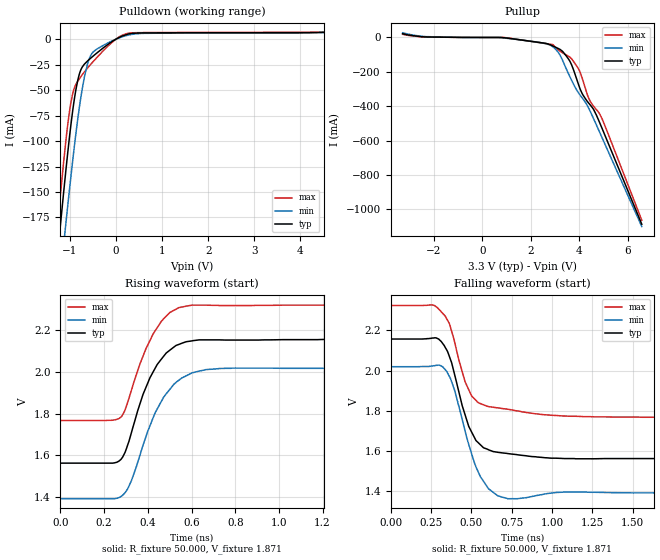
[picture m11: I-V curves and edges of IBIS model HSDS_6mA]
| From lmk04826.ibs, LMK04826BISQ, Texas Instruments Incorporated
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[Model]   HSDS_6mA
Model_type   Output
Polarity   Non-Inverting
Vmeas = 1.9
Vref = 1.9
Cref = 15pF
Rref = 50
|   typ   min   max
|   (nom PVT)   (Fast PVT)   (slow PVT)
C_comp   1.492p   1.392p   1.674p
|C_comp (hi state)   1.492p   1.392p   1.674p
|C_comp (low state)   2.777p   2.419p   2.781p
| Where   nom PVT is  Nominal Process, 3.3V, 27C
|   Fast PVT is Strong Process, 3.45V, -40C
|   Slow PVT is Weak Process, 3.15V, 125C
[Voltage Range]   3.3   3.15   3.45
[Temperature Range]   27   125   -40
[Pullup Reference]   3.3   3.15   3.45
[Pulldown Reference]   0   0   0
[Power Clamp Reference]   3.3   3.15   3.45
[GND Clamp Reference]   0   0   0
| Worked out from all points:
|   slope of the pulldown table from 0 to 0.495 V, typ, clamps not added: 81.8 ohm
|   slope of the pullup table from 0 to 0.495 V, typ, clamps not added: 8 kohm
|   falling waveform, R_fixture 50.000, V_fixture 1.871: 20-80 % time 131ps typ, 131ps min, 127ps max; typ from 2.16 V to 1.56 V
|   rising waveform, R_fixture 50.000, V_fixture 1.871: 20-80 % time 127ps typ, 145ps min, 127ps max; typ from 1.56 V to 2.16 V
[Pulldown]
|   Voltage   I(typ)   I(min)   I(max)
-3.3V     -1.225A    -1.2A      -1.253A
-1.28V    -220mA     -267.9mA   -190.8mA
-1.221V   -191.9mA   -241.5mA   -162.2mA
-1.122V   -146.4mA   -198mA     -116.6mA
-1.073V   -124.5mA   -176.5mA   -95.65mA
-993.3mV  -91.71mA   -143.1mA   -67.69mA
-864.6mV  -49.48mA   -92.41mA   -44.34mA
-755.7mV  -29.9mA    -56.55mA   -36.73mA
-607.2mV  -21.23mA   -23.33mA   -28.05mA
-409.2mV  -13.55mA   -9.712mA   -17.97mA
145.2mV   3.146mA    2.35mA     3.956mA
6.59V     8.158mA    8.228mA    8.143mA
[Pullup]
|   Voltage   I(typ)   I(min)   I(max)
-3.3V     22.29mA    27.13mA    18.75mA
-2.35V    3.194mA    4.974mA    2.65mA
887.7mV   -1.305mA   -2.825mA   -285.8uA
2.363V    -29.22mA   -28.44mA   -30.16mA
2.907V    -48.93mA   -53.53mA   -41.57mA
3.303V    -79.32mA   -129.3mA   -88.07mA
3.679V    -156.4mA   -246.4mA   -122.6mA
3.986V    -278.6mA   -324.7mA   -186.1mA
4.412V    -384.7mA   -416.3mA   -358.4mA
4.709V    -450.1mA   -507.4mA   -418.8mA
4.957V    -531.6mA   -585.6mA   -475.6mA
6.59V     -1.086A    -1.1A      -1.063A
[Ramp]
R_load = 50
|   typ   min   max
dV/dt_r   0.350058/1.26814e-10   0.377034/1.45031e-10   0.33351/1.26836e-10
dV/dt_f   0.350156/1.31831e-10   0.377034/1.30965e-10   0.333973/1.27082e-10
[Falling Waveform]
R_fixture = 50.000
V_fixture = 1.871
V_fixture_min = 1.682
V_fixture_max = 2.094
C_fixture = 0.000
|  time   V(typ)   V(min)   V(max)
0s        2.157V     2.019V     2.324V
259.3ps   2.162V     2.023V     2.327V
325ps     2.132V     2.017V     2.283V
363.8ps   2.071V     1.971V     2.235V
398.8ps   1.973V     1.896V     2.135V
461.7ps   1.779V     1.698V     1.944V
529ps     1.651V     1.52V      1.851V
606.1ps   1.605V     1.411V     1.82V
726.1ps   1.586V     1.361V     1.807V
3ns       1.562V     1.391V     1.767V
[Rising Waveform]
R_fixture = 50.000
V_fixture = 1.871
V_fixture_min = 1.682
V_fixture_max = 2.094
C_fixture = 0.000
|  time   V(typ)   V(min)   V(max)
0s        1.562V     1.391V     1.767V
240.4ps   1.562V     1.391V     1.769V
284.2ps   1.59V      1.407V     1.794V
325ps     1.709V     1.478V     1.913V
378.2ps   1.893V     1.648V     2.077V
443.3ps   2.037V     1.823V     2.214V
501.6ps   2.106V     1.918V     2.287V
531.4ps   2.129V     1.953V     2.304V
666.1ps   2.155V     2.012V     2.322V
3ns       2.157V     2.019V     2.323V
